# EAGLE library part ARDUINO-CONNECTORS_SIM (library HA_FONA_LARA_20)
SIM connector
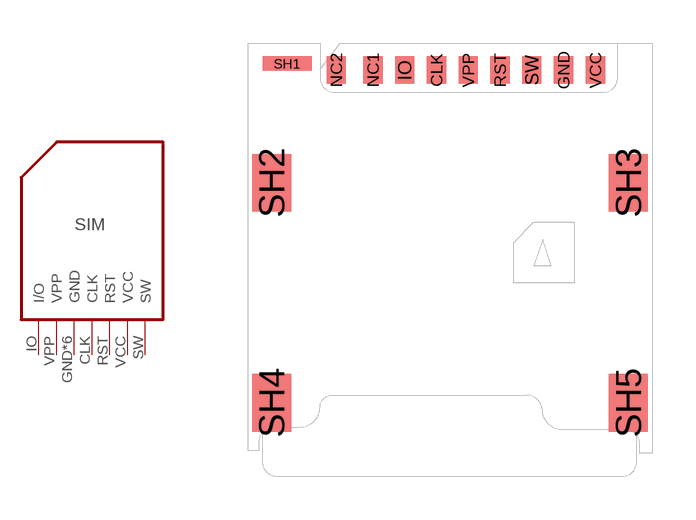
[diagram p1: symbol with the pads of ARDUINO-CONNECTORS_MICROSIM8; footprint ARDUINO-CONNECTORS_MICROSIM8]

Designator prefix SIM

## ARDUINO-CONNECTORS_SIM (CODE-BCE: -; CODE-TK2: -; DATASHEET: http://www.te.com/commerce/DocumentDelivery/DDEController?Action=srchrtrv&DocNm=2199337&DocType=Customer+Drawing&DocLang=English; DISTRIBUTOR-LINK: https://www.digikey.com/product-detail/en/te-connectivity-amp-connectors/2199337-5/A125065CT-ND/6810766; DISTRIBUTOR-PN: A125065CT-ND; MANUFACTURER: TE; MANUFACTURER-PN: 2199337-5; VALUE: -)  [ARDUINO-CONNECTORS_MICROSIM8]
CLK  CLK
GND  GND
IO  I/O
RST  RST
SH1  GND
SH2  GND
SH3  GND
SH4  GND
SH5  GND
SW  SW
VCC  VCC
VPP  VPP

## Footprint ARDUINO-CONNECTORS_MICROSIM8 (pad centres in mm)
smd 0.67 x 0.95: CLK -0.47,6.77; GND 3.93,6.77; IO -1.57,6.77; NC1 -2.67,6.77; NC2 -3.94,6.77; RST 1.73,6.77; SW 2.83,6.77; VCC 5.03,6.77; VPP 0.63,6.77
smd 1.7 x 0.5: SH1 -5.64,6.995
smd 1.35 x 2: SH2 -6.175,2.865; SH3 6.175,2.865; SH4 -6.175,-4.755; SH5 6.175,-4.755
